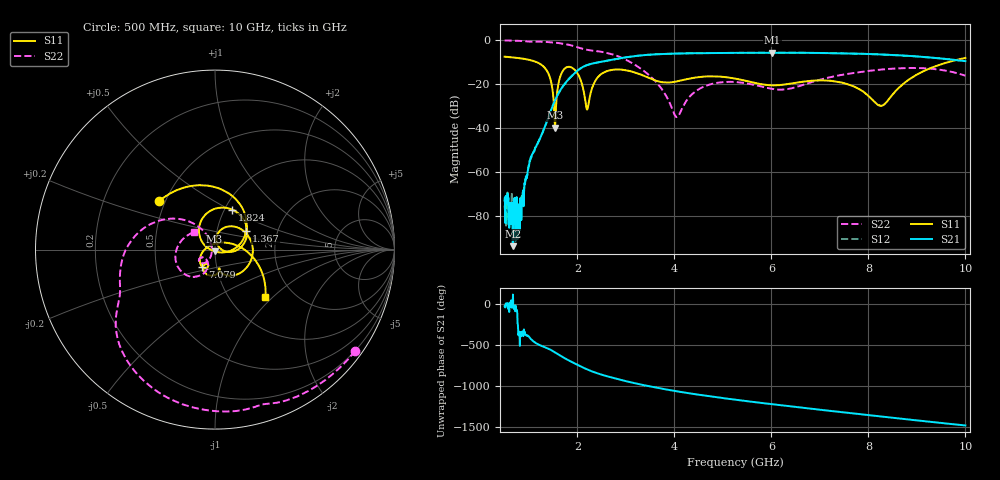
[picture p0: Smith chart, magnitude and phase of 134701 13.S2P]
!  2-Port S-parameters saved by WinCal
! VAR MeasName=S-Parameters (CALIBRATED_DATA) read from VNA (N5242A)
! VAR MeasDate=2013-7-3 16:29:24
! VAR NAME=134701 13
! VAR FILENAME=134701 13.S2P
! VAR DATE=2013-7-3 16:29:24
! VAR PHYS_PORTS=1,2
# Hz S MA R 50
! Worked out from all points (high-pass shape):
!   1601 points, 500 MHz to 10 GHz, reference 50 ohm
!   highest |S21| = -5.88 dB at 6.022 GHz (marker M1); lowest = -93.8 dB at 672.2 MHz (marker M2)
!   |S21| within 3 dB of the highest: 2.765 GHz to 9.648 GHz (6.883 GHz wide, 111 % of centre)
!   lowest |S11| = -39.9 dB at 1.539 GHz (marker M3), VSWR 1.02, Z = 49.7 - j0.964 ohm
!   |S11| at or under -10 dB: 1.14 GHz to 9.673 GHz (8.533 GHz wide, 158 % of centre)
!   |S22| runs from -35.2 to -0.3 dB; largest |S21 - S12| = 0.0029
!   S11 on the Smith chart (normalised r, x): 500 MHz: 0.46, +0.30; 1.367 GHz: 1.38, +0.30; 1.824 GHz: 1.09, +0.52; 7.079 GHz: 0.85, -0.17; 10 GHz: 1.45, -0.90
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5e8  0.412 139.2  0.0002207 -23.5  0.0001707 -45.9  0.963 -35.9
6.721875e8  0.3955 124.5  2.035e-05 120.4  0.0001152 -14.3  0.953 -48.1
8.028125e8  0.381 112.4  0.0001578 -21.1  0.0001762 -22.6  0.9418 -57.5
1.040312e9  0.3422 86.5  0.002152 -63.7  0.002069 -63.5  0.9025 -73.4
1.366875e9  0.2014 30.9  0.01332 -172.4  0.0134 -172.6  0.8893 -96.7
1.539062e9  0.01007 -105.9  0.04213 133.8  0.042 133.7  0.8599 -110.0
1.66375e9  0.1634 121.4  0.07594 88.4  0.07569 88.2  0.8272 -119.7
1.824062e9  0.243 66.4  0.1282 35.2  0.128 35.2  0.7684 -132.3
2.085312e9  0.1061 -5.2  0.2319 -42.4  0.2315 -42.4  0.6324 -149.2
2.21e9  0.02699 50.0  0.2679 -76.0  0.2675 -76.1  0.5869 -154.6
2.429688e9  0.1436 62.4  0.3063 -125.0  0.3057 -124.9  0.5451 -166.1
2.833438e9  0.2112 -6.2  0.3711 167.1  0.3712 167.1  0.4234 164.9
3.670625e9  0.1133 -78.8  0.4702 58.1  0.4697 58.1  0.09506 119.6
4.050625e9  0.1133 -76.4  0.4861 18.4  0.4859 18.3  0.01746 -179.3
4.507812e9  0.1417 -89.9  0.4949 -23.8  0.4954 -23.8  0.07558 -122.7
5.25e9  0.131 -120.1  0.5021 -83.7  0.5028 -83.7  0.1095 -144.6
6.021875e9  0.0923 -118.5  0.508 -139.6  0.5072 -139.7  0.07653 -142.5
6.835312e9  0.1169 -118.2  0.5033 164.6  0.5032 164.6  0.1093 -111.6
7.07875e9  0.1189 -126.3  0.4986 148.5  0.4993 148.3  0.13 -112.6
8.420625e9  0.04453 58.0  0.4548 60.7  0.4532 60.7  0.217 -140.8
9.032188e9  0.1686 -1.2  0.4145 21.1  0.4144 21.3  0.2274 -163.3
1e10  0.3851 -43.2  0.3263 -38.6  0.327 -38.3  0.1521 140.0
